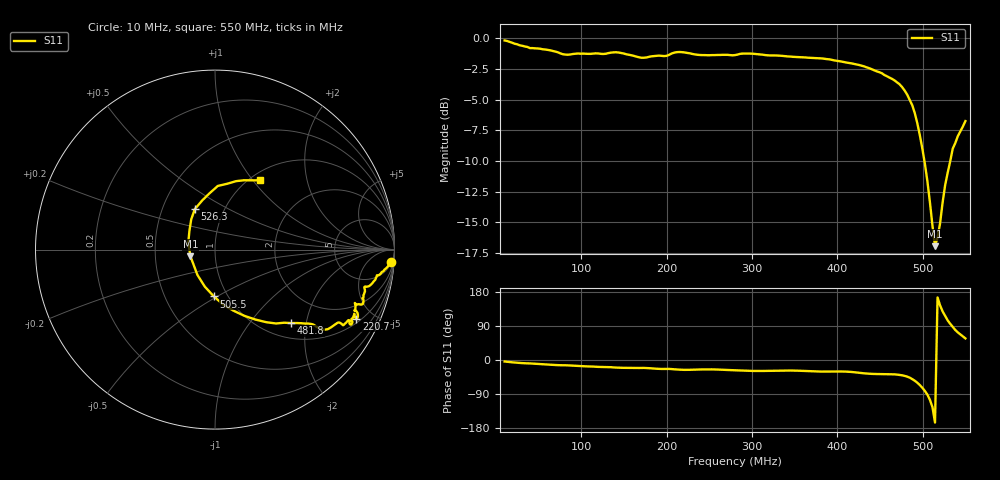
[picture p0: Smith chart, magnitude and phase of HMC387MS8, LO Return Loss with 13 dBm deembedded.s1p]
!Hittite Microwave Corporation
!12 Elizabeth Drive
!Chelmsford, MA 01824
!Tel: 978-250-3343
!Fax: 978-250-3373
!Device: HMC387MS8, 450-500 MHz, GaAs MMIC High IP3 Mixer in 8-lead plastic SMT package
!Misc: LO Return Loss with 13 dBm, Room
# MHZ S MA R 50
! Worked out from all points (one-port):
!   183 points, 10 MHz to 550 MHz, reference 50 ohm
!   lowest |S11| = -17.0 dB at 514.4 MHz (marker M1), VSWR 1.33, Z = 37.8 - j2.82 ohm
!   |S11| at or under -10 dB: 502 MHz to 532.3 MHz (30.32 MHz wide, 5.86 % of centre)
!   S11 on the Smith chart (normalised r, x): 10 MHz: 7, -27; 220.7 MHz: 1.20, -3.99; 481.8 MHz: 1.31, -1.64; 505.5 MHz: 0.86, -0.48; 526.3 MHz: 0.73, +0.35; 550 MHz: 1.11, +1.09
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10  0.981 -4.0
33.736  0.927 -8.7
78.242  0.862 -13.8
146.484  0.872 -20.6
173.187  0.834 -20.9
214.725  0.88 -25.5
220.659  0.877 -26.0
250.33  0.854 -24.7
280  0.855 -27.2
303.736  0.864 -28.9
348.242  0.841 -27.9
377.912  0.83 -30.5
416.484  0.791 -31.6
440.22  0.749 -36.6
466.923  0.674 -37.9
475.824  0.633 -40.4
481.758  0.59 -43.9
484.725  0.561 -46.6
493.626  0.451 -59.9
499.56  0.355 -73.3
505.495  0.261 -91.4
511.429  0.172 -124.6
514.396  0.142 -165.1
520.33  0.176 144.2
526.264  0.252 116.5
535.165  0.355 87.5
541.099  0.399 72.9
550  0.46 57.0
